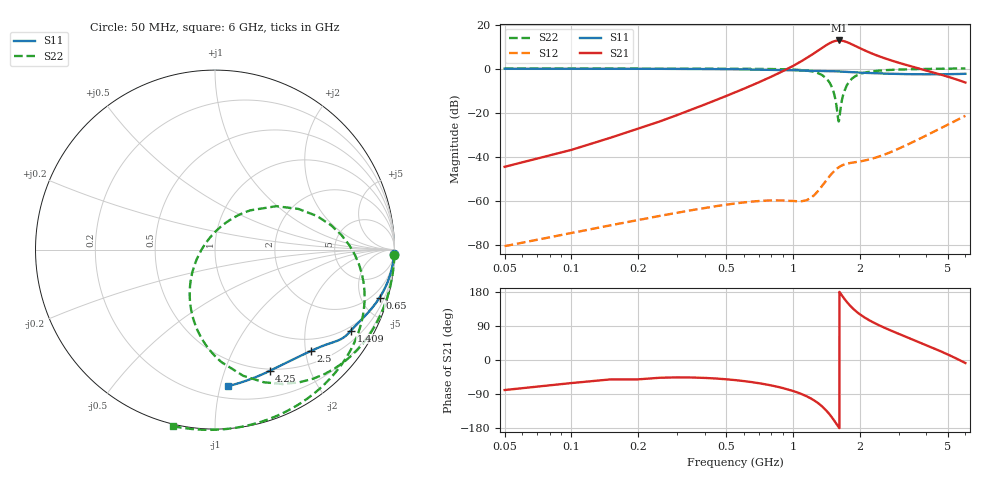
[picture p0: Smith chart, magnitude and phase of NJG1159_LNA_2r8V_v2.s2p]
! Created Mon Mar 05 15:35:13 2018
# hz S ma R 50
! 2 Port Network Data from SP6.SP block
! freq  magS11  angS11  magS21  angS21  magS12  angS12  magS22  angS22
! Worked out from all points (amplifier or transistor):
!   414 points, 50 MHz to 6 GHz, reference 50 ohm
!   highest |S21| = 12.8 dB at 1.615 GHz (marker M1)
!   |S21| within 3 dB of that: 1.372 GHz to 1.958 GHz (586 MHz wide, 35.2 % of centre)
!   unconditionally stable (mu >= 1): 503.6 MHz to 2.554 GHz
!   at 1.442 GHz: K = 6.83, MAG = 19.1 dB, |S12| = -49.7 dB
!   at 1.58 GHz: K = 5.27, MAG = 18.9 dB, |S12| = -45.4 dB
!   at 6 GHz: K = -0.81, MSG = 7.6 dB, |S12| = -21.4 dB
!   lowest NFmin = 0.14 dB at 100 MHz
!   S11 on the Smith chart (normalised r, x): 50 MHz: 12, -84; 650 MHz: 1.12, -6.81; 1.409 GHz: 0.85, -3.44; 2.5 GHz: 0.74, -2.10; 4.25 GHz: 0.48, -1.44; 6 GHz: 0.29, -1.06
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5e7  0.9968 -1.3  0.005875 -79.3  9.243e-05 87.9  1 -1.7
1.5e8  0.9944 -4.0  0.02683 -51.2  0.0002749 85.2  0.9997 -5.0
2.5e8  0.9898 -6.6  0.06275 -46.9  0.0004493 82.4  0.9989 -8.4
5.5e8  0.9654 -14.0  0.2909 -53.1  0.0008647 72.7  0.9935 -19.3
6.5e8  0.955 -16.3  0.4139 -58.3  0.0009502 68.5  0.9897 -23.3
1e9  0.916 -23.5  1.149 -81.7  0.0009844 36.6  0.9527 -41.3
1.15e9  0.9009 -26.2  1.727 -95.4  0.001021 -1.3  0.9033 -52.8
1.25e9  0.8924 -27.9  2.26 -107.0  0.001348 -34.7  0.8381 -63.3
1.4e9  0.8826 -30.6  3.312 -130.6  0.002708 -77.0  0.6313 -86.4
1.402e9  0.8825 -30.7  3.327 -131.0  0.002734 -77.5  0.6272 -86.8
1.409e9  0.8821 -30.8  3.38 -132.3  0.002825 -79.3  0.6126 -88.2
1.503e9  0.8759 -32.7  4.032 -152.3  0.004208 -102.0  0.365 -111.2
1.562e9  0.8703 -33.9  4.291 -166.2  0.005102 -115.7  0.1743 -135.8
1.615e9  0.8637 -35.0  4.368 -178.8  0.005801 -127.3  0.06663 124.2
1.698e9  0.8514 -36.5  4.213 163.2  0.006588 -142.9  0.2891 48.6
1.7e9  0.8511 -36.6  4.206 162.8  0.006603 -143.2  0.2945 48.0
1.9e9  0.8235 -39.5  3.326 131.5  0.007462 -165.5  0.6604 11.9
2.15e9  0.7996 -42.6  2.482 108.9  0.008359 -175.4  0.8285 -9.2
2.5e9  0.7769 -46.7  1.836 89.1  0.01046 -178.5  0.9095 -26.0
2.75e9  0.7653 -49.5  1.56 78.4  0.01258 -179.0  0.9356 -34.6
4.25e9  0.7417 -65.8  0.8309 32.7  0.03536 174.9  0.9893 -70.6
6e9  0.7634 -84.4  0.4829 -8.0  0.08479 160.4  1.011 -103.3
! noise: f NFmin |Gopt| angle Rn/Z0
5e+07  0.547  0.9625  2.486  3.5
1.418e+09  0.5129  0.8178  33.22  0.5179
1.464e+09  0.5243  0.8134  34.24  0.5132
1.51e+09  0.536  0.8089  35.26  0.5085
1.556e+09  0.5479  0.8044  36.28  0.5038
1.602e+09  0.56  0.7998  37.29  0.4992
1.648e+09  0.5723  0.7951  38.3  0.4945
1.694e+09  0.5848  0.7904  39.31  0.4899
3.7e+09  1.35  0.5488  76.83  0.3338
6e+09  3.169  0.434  83.8  0.6154
